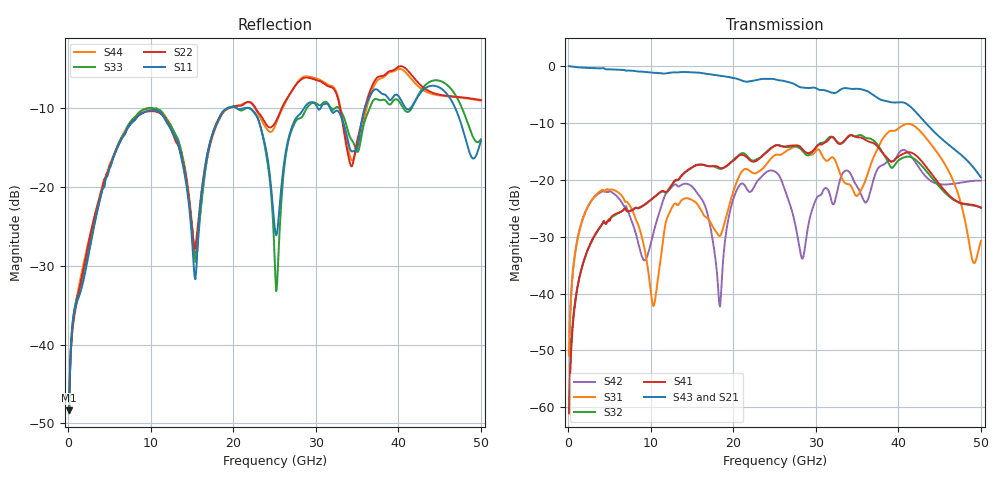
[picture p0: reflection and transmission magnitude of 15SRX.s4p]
! DAC39RF10ACK
! 256-pin FCBGA package
! Texas Instruments 8/20/2022
! Single-ended  S-parameters
! PORT#  PORT_NAME  NET_NAME
! PORT1:  xSRXN.DIEBUMP  xSRXN
! PORT2:  xSRXN.BGA  xSRXN
! PORT3:  xSRXP.DIEBUMP  xSRXP
! PORT4:  xSRXP.BGA  xSRXP
! Touchstone Ver. 1.0
! Number of ports is 4
# Hz	S	MA	R	50.000000
! SCATTERING PARAMETERS  :
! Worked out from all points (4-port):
!   500 points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, 100 MHz to 50 GHz, reference 50 ohm
!   strongest paths, dB at 100 MHz, 12.6 GHz, 25.1 GHz, 37.6 GHz, 50 GHz:
!     S43: 0.0, -1.1, -2.4, -5.7, -19.6
!     S21: 0.0, -1.1, -2.4, -6.3, -19.6
!     S41: -61.1, -20.8, -14.0, -14.3, -24.9
!     S32: -61.0, -20.9, -14.0, -14.1, -24.9
!     S31: -51.0, -24.8, -15.6, -14.2, -30.8
!     S42: -50.6, -21.2, -18.6, -17.9, -20.2
!   lowest |S11| = -48.3 dB at 100 MHz (marker M1), VSWR 1.01, Z = 50.3 + j0.214 ohm
!   |S11| at or under -10 dB: start of sweep to 19.28 GHz; 21.98 GHz to 28.55 GHz (6.569 GHz wide, 26 % of centre); 31.74 GHz to 35.91 GHz (4.174 GHz wide, 12.3 % of centre)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
1e8  0.003835 33.7  0.9958 -2.3  0.002781 85.5  0.0007186 -90.2
     0.9964 -2.2  0.003841 29.2  0.000851 -97.0  0.002898 85.5
     0.002817 85.4  0.0008896 -95.4  0.00366 32.3  0.9957 -2.2
     0.0008849 -97.3  0.002937 85.3  0.9967 -2.1  0.004101 31.6
3.1e9  0.05553 43.4  0.9588 -61.0  0.07017 25.6  0.03126 -159.7
       0.9581 -60.9  0.06243 -9.3  0.0319 -159.3  0.07009 28.4
       0.07022 25.5  0.03125 -159.4  0.05686 41.5  0.9555 -61.1
       0.03166 -159.3  0.0697 28.2  0.9572 -60.9  0.0628 -8.9
9e9  0.2954 -68.5  0.8884 -174.2  0.02919 -101.7  0.05865 84.5
     0.8915 -174.2  0.2952 -103.2  0.05849 85.0  0.02103 -141.4
     0.02971 -101.0  0.05913 85.6  0.309 -68.3  0.8926 -174.0
     0.05852 84.8  0.02051 -138.6  0.8914 -174.0  0.3048 -102.7
1.83e10  0.2754 -79.2  0.8165 6.6  0.0318 168.2  0.128 -95.9
         0.8165 6.5  0.2767 -91.3  0.1255 -94.0  0.007707 18.3
         0.032 170.1  0.1251 -93.3  0.2712 -79.7  0.8197 6.8
         0.1278 -96.5  0.008053 17.4  0.8209 6.8  0.2696 -90.5
2.71e10  0.2407 -50.3  0.7137 -165.2  0.1911 -136.3  0.1993 87.3
         0.7112 -165.3  0.4087 -117.4  0.1969 87.9  0.05251 -58.5
         0.1901 -136.6  0.197 88.2  0.2326 -59.0  0.7048 -165.2
         0.1998 87.0  0.0533 -60.0  0.7087 -165.3  0.409 -116.0
3.62e10  0.3461 -86.4  0.5686 14.2  0.1083 -154.5  0.2191 -112.5
         0.5748 14.2  0.3569 -111.2  0.2335 -111.6  0.06468 -150.6
         0.1078 -154.6  0.2319 -111.0  0.2877 -89.8  0.5948 17.0
         0.2198 -113.3  0.06449 -151.5  0.6025 17.0  0.3252 -111.0
5e10  0.1962 -95.0  0.1007 129.2  0.02897 -2.3  0.067 10.5
      0.1045 123.1  0.3577 -169.1  0.041 8.2  0.09566 26.9
      0.02896 -0.5  0.05689 12.9  0.201 -113.8  0.09171 128.7
      0.05687 4.9  0.09824 25.5  0.105 118.6  0.3541 -167.8
